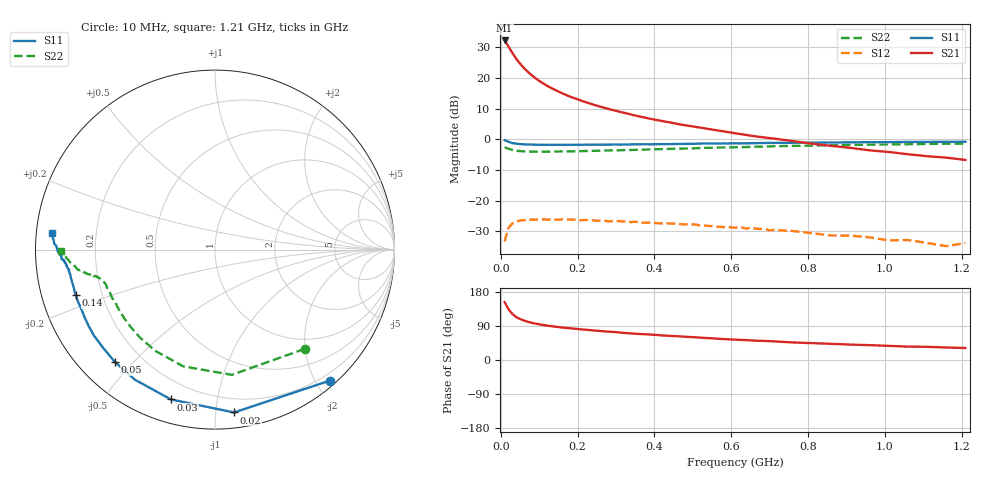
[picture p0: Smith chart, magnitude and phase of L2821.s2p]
!  POLYFET RF DEVICES
!  L2821 S-PARAMETERS
!  Vds=12.5V,Idq=200ma,Vgs=3.08V
# MHZ S MA R 50
! Freq=MHz Mag[s11] Ang[s11] Mag[s21] Ang[s21] Mag[s12] Ang[s12] Mag[s22] Ang[s22]
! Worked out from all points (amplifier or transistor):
!   81 points, 10 MHz to 1.21 GHz, reference 50 ohm
!   highest |S21| = 32.2 dB at 10 MHz (marker M1)
!   |S21| within 3 dB of that: start of sweep to 25.05 MHz
!   unconditionally stable (mu >= 1): 819 MHz to end of sweep
!   at 140 MHz: K = 0.14, MSG = 21.2 dB, |S12| = -26.2 dB
!   at 410 MHz: K = 0.47, MSG = 16.8 dB, |S12| = -27.3 dB
!   at 1.21 GHz: K = 1.66, MAG = 8.8 dB, |S12| = -33.8 dB
!   S11 on the Smith chart (normalised r, x): 10 MHz: 0.09, -2.20; 20 MHz: 0.10, -1.12; 30 MHz: 0.11, -0.74; 50 MHz: 0.11, -0.44; 140 MHz: 0.10, -0.16; 1.21 GHz: 0.04, +0.05
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10  0.9702 -48.8  40.88 152.8  0.02175 65.8  0.7452 -47.9
20  0.9136 -83.3  32.62 134.0  0.03606 44.6  0.7041 -82.3
30  0.8702 -106.4  25.73 121.7  0.04256 32.1  0.6743 -105.3
40  0.8512 -121.6  20.61 113.4  0.04567 23.9  0.6548 -120.5
50  0.8386 -131.7  17.21 108.3  0.04767 19.2  0.6442 -130.4
60  0.8292 -139.1  14.62 104.2  0.04828 15.3  0.6376 -137.5
70  0.8273 -144.8  12.67 101.0  0.0489 12.0  0.6344 -142.9
80  0.8225 -148.8  11.19 98.2  0.04939 10.1  0.6318 -146.8
90  0.8189 -152.2  9.981 96.1  0.04918 7.9  0.6301 -150.0
100  0.8161 -154.7  8.977 94.2  0.04974 6.2  0.6278 -152.4
110  0.8151 -156.9  8.189 92.5  0.04973 4.5  0.6326 -154.5
140  0.816 -161.9  6.456 88.2  0.04925 1.5  0.6336 -158.6
170  0.8151 -165.0  5.275 84.7  0.04957 -2.1  0.638 -161.2
210  0.817 -168.3  4.257 80.8  0.04812 -4.6  0.6432 -163.4
250  0.818 -170.1  3.543 77.3  0.04702 -6.8  0.6521 -164.9
290  0.8221 -171.5  3.022 74.3  0.04658 -9.4  0.6616 -165.9
350  0.8293 -173.4  2.447 69.4  0.04553 -12.6  0.6752 -166.9
410  0.8352 -174.5  2.045 65.8  0.04298 -14.4  0.6905 -167.9
610  0.8644 -178.4  1.259 53.8  0.03625 -20.4  0.7443 -170.3
810  0.8834 178.9  0.8514 44.5  0.02969 -22.4  0.7899 -173.8
1010  0.9014 176.5  0.6237 37.3  0.02263 -19.0  0.8273 -176.6
1210  0.9146 174.0  0.4623 31.7  0.02045 -6.0  0.8553 -179.3
